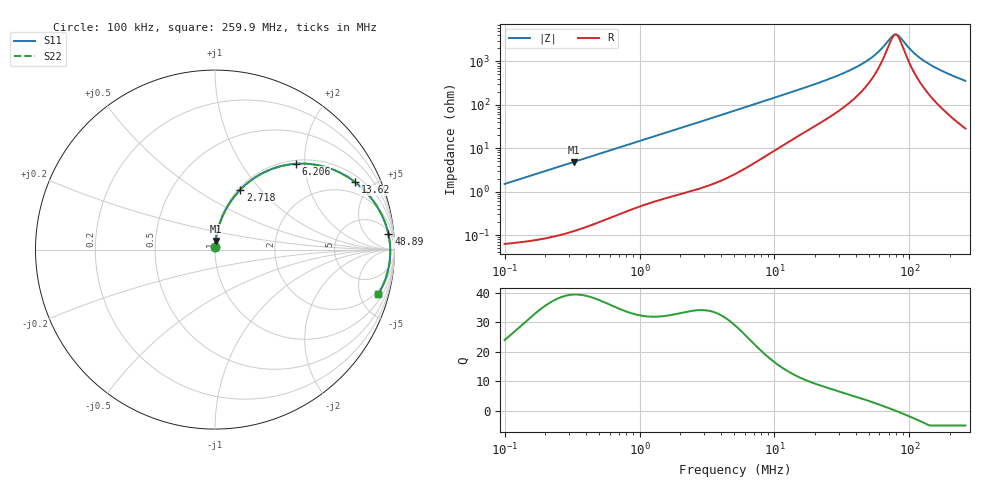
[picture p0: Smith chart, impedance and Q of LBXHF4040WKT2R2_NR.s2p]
! LBXHF4040WKT2R2_NR  S-PARAMETER MODEL  ( General Type )
! Model Generated by TAIYO YUDEN Corporation (http://www.ty-top.com)
! Version 1.0
! TAIYO YUDEN Control No. 210719NI43SB-FBB
! Copyright(c) 2021 TAIYO YUDEN CO.,LTD. All Rights Reserved.
! Product Description (link to TY-COMPAS)
! https://ds.yuden.co.jp/TYCOMPAS/or/detail?pn=LBXHF4040WKT2R2MNR&u=M
! Products Name : Inductors
! Characteristics :
!  Inductance : 2.2 uH , SRF(min) : 55 MHz , DC Resistance(max) : 0.052 Ohm
!  Rated Current : Saturation :3000 mA , Temp Rise : 1910 mA
!  Case Size : 4.0 x 4.0 / 0.157 x 0.157 [mm/inch] , Thickness : 2 / 0.079 [mm/inch]
!  (Conditions: Temperature = 25 degC , DC Bias Current/Voltage = 0A / 0V)
! External Node Assignments :
!  1  o---GGG---o  2
! GND o---------o GND
! Frequency Range : 0.1MHz  -  259.929867MHz  [ 402 STEP ]
# MHz S RI R 50
! Freq[MHz].  S11 Real  S11 Imag  S21 Real  S21 Imag  S12 Real  S12 Imag  S22 Real  S22 Imag
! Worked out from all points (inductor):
!   401 points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, 100 kHz to 259.9 MHz, reference 50 ohm
!   read as one part in series: L = 2.39 uH near 104 kHz
!   highest Q = 39.4 at 325.3 kHz (marker M1), where L = 2.38 uH
!   self-resonance near 78.86 MHz
!   S11 on the Smith chart (normalised r, x): 100 kHz: 1.00, +0.03; 2.718 MHz: 1.02, +0.79; 6.206 MHz: 1.07, +1.80; 13.62 MHz: 1.32, +3.99; 48.89 MHz: 7, +20; 259.9 MHz: 1.57, -7.09
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0.1  0.000855 0.015  0.9991 -0.015  0.9991 -0.015  0.000855 0.015
0.325258  0.00359 0.0484  0.9964 -0.0484  0.9964 -0.0484  0.00359 0.0484
0.37324  0.00451 0.0554  0.9955 -0.0554  0.9955 -0.0554  0.00451 0.0554
0.7574  0.0156 0.11  0.9844 -0.11  0.9844 -0.11  0.0156 0.11
1.393082  0.0453 0.193  0.9547 -0.193  0.9547 -0.193  0.0453 0.193
2.717938  0.141 0.3337  0.859 -0.3337  0.859 -0.3337  0.141 0.3337
3.722493  0.2312 0.4068  0.7688 -0.4068  0.7688 -0.4068  0.2312 0.4068
5.098332  0.3573 0.4622  0.6427 -0.4622  0.6427 -0.4622  0.3573 0.4622
6.205825  0.4495 0.478  0.5505 -0.478  0.5505 -0.478  0.4495 0.478
8.840321  0.6175 0.4596  0.3825 -0.4596  0.3825 -0.4596  0.6175 0.4596
13.62339  0.7819 0.3748  0.2181 -0.3748  0.2181 -0.3748  0.7819 0.3748
19.02902  0.8657 0.2925  0.1343 -0.2925  0.1343 -0.2925  0.8657 0.2925
32.99563  0.9418 0.165  0.0582 -0.165  0.0582 -0.165  0.9418 0.165
48.88766  0.9664 0.0865  0.0336 -0.0865  0.0336 -0.0865  0.9664 0.0865
59.50735  0.9727 0.0503  0.0273 -0.0503  0.0273 -0.0503  0.9727 0.0503
71.02397  0.9758 0.0186  0.0242 -0.0186  0.0242 -0.0186  0.9758 0.0186
76.83401  0.9764 0.00463  0.0236 -0.00463  0.0236 -0.00463  0.9764 0.00463
81.50137  0.9766 -0.00586  0.0234 0.00586  0.0234 0.00586  0.9766 -0.00586
107.321  0.9741 -0.0557  0.0259 0.0557  0.0259 0.0557  0.9741 -0.0557
130.634  0.9686 -0.0932  0.0314 0.0932  0.0314 0.0932  0.9686 -0.0932
178.9166  0.9513 -0.1591  0.0487 0.1591  0.0487 0.1591  0.9513 -0.1591
259.9299  0.9098 -0.2493  0.0902 0.2493  0.0902 0.2493  0.9098 -0.2493
